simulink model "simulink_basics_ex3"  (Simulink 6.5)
settings: Solver=VariableStepDiscrete  StartTime=0.0  StopTime=10  FixedStep=Tsample  RelTol=1e-3

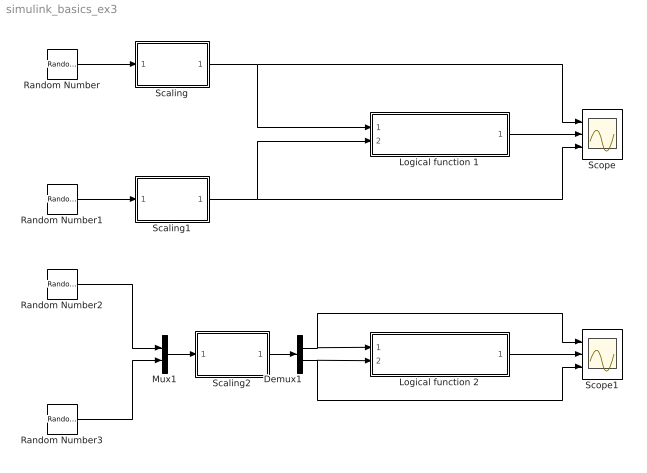
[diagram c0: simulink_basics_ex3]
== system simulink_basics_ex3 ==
  Demux1 : Demux  Outputs=2
  Logical function 1 : Subsystem
  Logical function 2 : Subsystem
  Mux1 : Mux  Inputs=2
  Random Number : RandomNumber  SampleTime=0
  Random Number1 : RandomNumber  Seed=1  SampleTime=0
  Random Number2 : RandomNumber  SampleTime=0
  Random Number3 : RandomNumber  Seed=1  SampleTime=0
  Scaling : Subsystem
  Scaling1 : Subsystem
  Scaling2 : Subsystem
  Scope : Scope  NumInputPorts=3
  Scope1 : Scope  NumInputPorts=3
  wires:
  Logical function 1/1(y) -> Scope/2
  Random Number1/1 -> Scaling1/1(In1)
  Logical function 2/1(y) -> Scope1/2
  Random Number2/1 -> Mux1/1
  Random Number3/1 -> Mux1/2
  Scaling2/1(Out1) -> Demux1/1
  Demux1/1 -> Logical function 2/1(A), Scope1/1
  Demux1/2 -> Logical function 2/2(B), Scope1/3
  Mux1/1 -> Scaling2/1(In1)
  Scaling/1(Out1) -> Scope/1, Logical function 1/1(A)
  Scaling1/1(Out1) -> Scope/3, Logical function 1/2(B)
  Random Number/1 -> Scaling/1(In1)

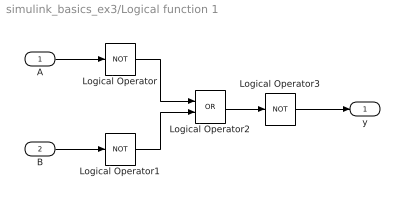
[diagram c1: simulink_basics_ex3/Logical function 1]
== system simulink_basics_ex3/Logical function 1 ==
  A : Inport
  B : Inport  Port=2
  Logical Operator : Logic  Operator=NOT  AllPortsSameDT=off  OutDataTypeMode=Boolean
  Logical Operator1 : Logic  Operator=NOT  AllPortsSameDT=off  OutDataTypeMode=Boolean
  Logical Operator2 : Logic  Operator=OR  AllPortsSameDT=off  OutDataTypeMode=Boolean
  Logical Operator3 : Logic  Operator=NOT  AllPortsSameDT=off  OutDataTypeMode=Boolean
  y : Outport
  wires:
  Logical Operator/1 -> Logical Operator2/1
  Logical Operator1/1 -> Logical Operator2/2
  Logical Operator2/1 -> Logical Operator3/1
  A/1 -> Logical Operator/1
  Logical Operator3/1 -> y/1
  B/1 -> Logical Operator1/1

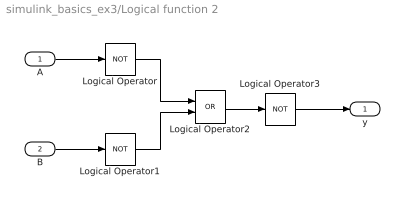
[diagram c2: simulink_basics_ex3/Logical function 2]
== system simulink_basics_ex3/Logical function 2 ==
  A : Inport
  B : Inport  Port=2
  Logical Operator : Logic  Operator=NOT  AllPortsSameDT=off  OutDataTypeMode=Boolean
  Logical Operator1 : Logic  Operator=NOT  AllPortsSameDT=off  OutDataTypeMode=Boolean
  Logical Operator2 : Logic  Operator=OR  AllPortsSameDT=off  OutDataTypeMode=Boolean
  Logical Operator3 : Logic  Operator=NOT  AllPortsSameDT=off  OutDataTypeMode=Boolean
  y : Outport
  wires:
  B/1 -> Logical Operator1/1
  Logical Operator3/1 -> y/1
  A/1 -> Logical Operator/1
  Logical Operator2/1 -> Logical Operator3/1
  Logical Operator1/1 -> Logical Operator2/2
  Logical Operator/1 -> Logical Operator2/1

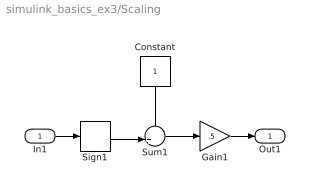
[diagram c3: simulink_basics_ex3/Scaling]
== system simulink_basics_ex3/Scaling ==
  In1 : Inport
  Constant : Constant  Orientation=down  Value=1  OutDataType=sfix(16)  ConRadixGroup=Use specified scaling  OutScaling=2^0  SampleTime=inf  FramePeriod=inf
  Gain1 : Gain  Gain=.5
  Sign1 : Signum
  Sum1 : Sum  Inputs=++|
  Out1 : Outport
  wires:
  Sign1/1 -> Sum1/2
  Sum1/1 -> Gain1/1
  Constant/1 -> Sum1/1
  Gain1/1 -> Out1/1
  In1/1 -> Sign1/1

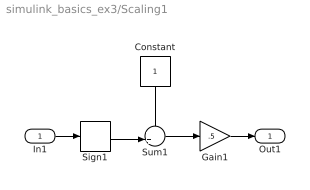
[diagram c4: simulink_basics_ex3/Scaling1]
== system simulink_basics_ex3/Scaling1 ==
  In1 : Inport
  Constant : Constant  Orientation=down  Value=1  OutDataType=sfix(16)  ConRadixGroup=Use specified scaling  OutScaling=2^0  SampleTime=inf  FramePeriod=inf
  Gain1 : Gain  Gain=.5
  Sign1 : Signum
  Sum1 : Sum  Inputs=++|
  Out1 : Outport
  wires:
  In1/1 -> Sign1/1
  Gain1/1 -> Out1/1
  Constant/1 -> Sum1/1
  Sum1/1 -> Gain1/1
  Sign1/1 -> Sum1/2

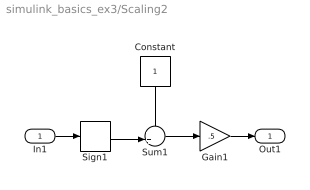
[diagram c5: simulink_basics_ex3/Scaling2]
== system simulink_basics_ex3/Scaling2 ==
  In1 : Inport
  Constant : Constant  Orientation=down  Value=1  OutDataType=sfix(16)  ConRadixGroup=Use specified scaling  OutScaling=2^0  SampleTime=inf  FramePeriod=inf
  Gain1 : Gain  Gain=.5
  Sign1 : Signum
  Sum1 : Sum  Inputs=++|
  Out1 : Outport
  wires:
  In1/1 -> Sign1/1
  Gain1/1 -> Out1/1
  Constant/1 -> Sum1/1
  Sum1/1 -> Gain1/1
  Sign1/1 -> Sum1/2
